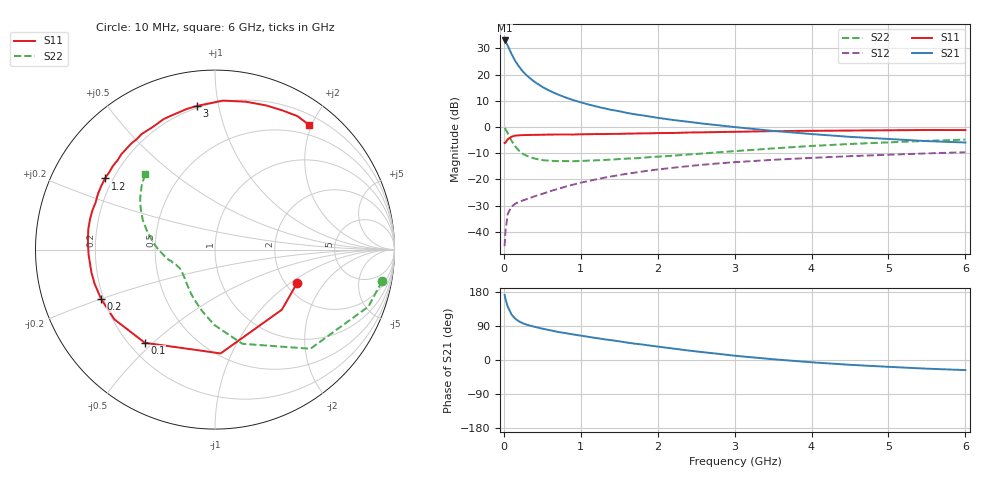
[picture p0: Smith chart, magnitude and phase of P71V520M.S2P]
! SIEMENS Small Signal Semiconductors
! BFP196
! Si NPN RF Bipolar Junction Transistor in SOT143
! VCE = 1.5 V  IC = 20 mA
! Common Emitter S-Parameters:  May  1996
# GHz  S  MA  R  50
!  f  S11  S21  S12  S22
! GHz  MAG  ANG  MAG  ANG  MAG  ANG  MAG  ANG
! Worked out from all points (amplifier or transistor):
!   36 points, 10 MHz to 6 GHz, reference 50 ohm
!   highest |S21| = 33.0 dB at 10 MHz (marker M1)
!   |S21| within 3 dB of that: start of sweep to 66.37 MHz
!   unconditionally stable (mu >= 1): 649.7 MHz to 3.418 GHz; 3.998213 GHz to 4.002516 GHz
!   at 250 MHz: K = 0.61, MSG = 24.5 dB, |S12| = -28.0 dB
!   at 1.4 GHz: K = 1.12, MAG = 10.6 dB, |S12| = -18.9 dB
!   at 6 GHz: K = 0.99, MSG = 1.9 dB, |S12| = -9.7 dB
!   S11 on the Smith chart (normalised r, x): 10 MHz: 2.30, -1.13; 100 MHz: 0.26, -0.47; 200 MHz: 0.19, -0.20; 1.2 GHz: 0.17, +0.29; 3 GHz: 0.19, +0.87; 6 GHz: 0.34, +1.97
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0.01  0.4942 -22.2  44.64 171.5  0.0053 82.7  0.9472 -10.7
0.02  0.5008 -42.0  42.57 162.1  0.0098 76.4  0.9117 -20.4
0.05  0.5793 -86.9  35.66 141.1  0.0216 57.9  0.7667 -46.1
0.1  0.65 -127.0  24.66 120.0  0.0302 44.1  0.5463 -73.8
0.15  0.6822 -145.3  17.92 108.7  0.0343 40.2  0.42 -90.5
0.2  0.6918 -156.6  13.98 101.5  0.0371 39.5  0.3492 -102.0
0.25  0.6974 -164.2  11.31 96.6  0.0397 40.0  0.3046 -111.6
0.3  0.7001 -169.6  9.517 93.1  0.042 41.6  0.28 -118.4
0.4  0.7051 -177.8  7.237 87.5  0.0474 44.4  0.2483 -128.9
0.5  0.7093 176.6  5.801 82.8  0.0528 47.5  0.2326 -136.3
0.6  0.7148 171.1  4.849 78.5  0.0592 49.3  0.2257 -141.8
0.7  0.7166 166.2  4.177 74.3  0.0654 51.0  0.2229 -145.7
0.9  0.7151 158.5  3.256 67.6  0.0792 51.9  0.2216 -151.6
1.1  0.726 150.7  2.679 61.1  0.0926 52.4  0.2274 -155.6
1.2  0.73 147.1  2.463 58.0  0.0997 52.2  0.2305 -157.5
1.7  0.7484 130.9  1.744 43.1  0.1339 48.6  0.2515 -165.3
2.2  0.7658 117.1  1.357 30.2  0.1664 43.1  0.2825 -172.4
3  0.8069 97.1  0.993 11.3  0.2124 33.0  0.345 173.8
3.5  0.8313 87.0  0.839 2.0  0.2357 26.7  0.3885 165.5
4.5  0.8524 70.4  0.646 -12.7  0.2765 15.3  0.4723 151.2
5.5  0.874 58.3  0.536 -22.9  0.3124 4.4  0.5422 138.9
6  0.8705 52.8  0.504 -26.6  0.3287 -1.5  0.573 132.9
